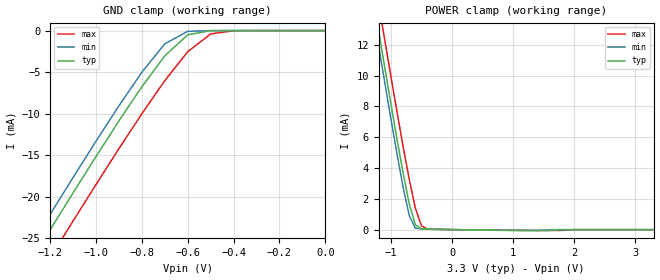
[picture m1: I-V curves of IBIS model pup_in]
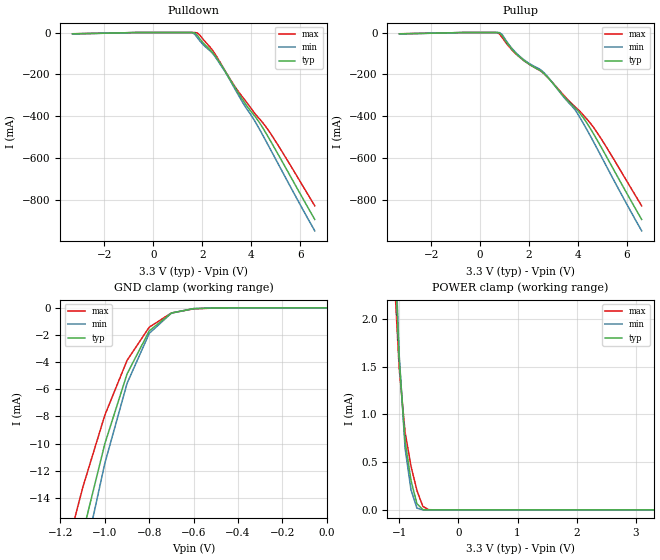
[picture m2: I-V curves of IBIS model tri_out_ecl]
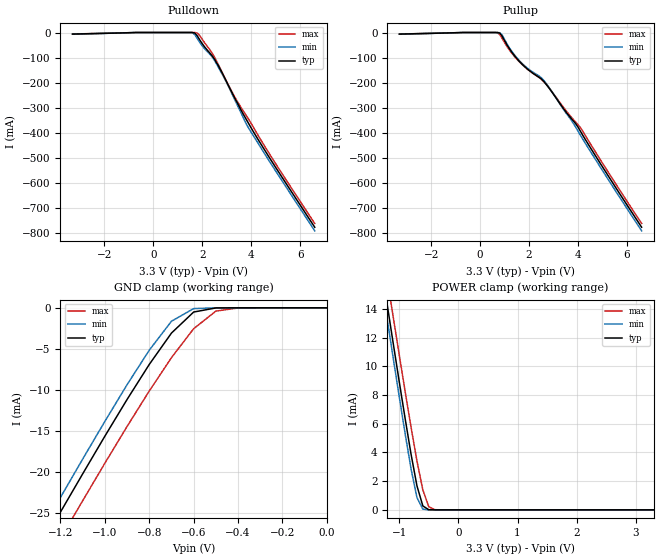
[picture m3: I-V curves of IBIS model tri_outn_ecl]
| IBIS file EG2101CA.ibs
[IBIS ver]   3.2
[File name]   eg2101ca.ibs
[File Rev]   2
[Date]   December 26, 2006
[Source]   Circuits Simulation by HSPICE.
|   Component EG-2101CA
[Component]   EG-2101CA
[Manufacturer]   Epson Toyocom Corp.
[Package]
| variable   typ   min   max
R_pkg   1.04   NA   NA
L_pkg   1.98nH  NA   NA
C_pkg   3.71pF  NA   NA
[Pin]   signal_name   model_name   R_pin   L_pin   C_pin
1   oe   pup_in   NA   NA   NA
4   out   tri_out_ecl   NA   NA   NA
5   outn   tri_outn_ecl   NA   NA   NA
6   vdd   POWER   NA   NA   NA
3   vss   GND   NA   NA   NA
[Diff Pin] inv_pin vdiff   tdelay_typ
4   5   0   0
| Models and submodels in the file (3): pup_in (Input), tri_out_ecl (3-state_ECL), tri_outn_ecl (3-state_ECL)
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|   Model pup_in
[Model]   pup_in
Model_type   Input
C_comp   1.00pF  0.70pF  1.43pF
Vinl = 0.99V | VIL = VCC * 0.3
Vinh = 2.31V | VIH = VCC * 0.7
|   typ   min   max
[Temperature Range]   25.00  0.000  70.00
[Voltage Range]   3.30V  3.00V  3.60V
[POWER Clamp Reference]   3.30V  3.00V  3.60V
[GND Clamp Reference]   0.00V  0.00V  0.00V
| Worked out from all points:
|   GND clamp passes 1 mA (typ) near -0.62 V on its own axis
|   POWER clamp passes 1 mA (typ) near -0.65 V on its own axis
[GND_clamp]
| voltage = voutput
| voltage   I(typ)   I(min)   I(max)
-3.3V     -120.5mA   -118.7mA   -123.7mA
-1.3V     -28.46mA   -26.61mA   -31.84mA
-1.2V     -23.98mA   -22.12mA   -27.37mA
-1.1V     -19.54mA   -17.68mA   -22.92mA
-900mV    -10.87mA   -9.048mA   -14.21mA
-800mV    -6.758mA   -5.013mA   -10.01mA
-700mV    -3.036mA   -1.593mA   -6.026mA
-600mV    -509.4uA   -93.51uA   -2.539mA
-500mV    -21.23uA   -6.595uA   -406.6uA
-400mV    -6.143uA   -5.249uA   -23.62uA
0V        -5.82uA    -5.224uA   -5.655uA
[POWER_clamp]
| voltage = vcc - voutput
| voltage   I(typ)   I(min)   I(max)
-3.3V     64.56mA    63.65mA    66.23mA
-1.3V     15.28mA    14.3mA     17.06mA
-1.2V     12.88mA    11.9mA     14.67mA
-1.1V     10.5mA     9.52mA     12.29mA
-900mV    5.86mA     4.896mA    7.632mA
-800mV    3.66mA     2.731mA    5.38mA
-700mV    1.667mA    901.9uA    3.253mA
-600mV    312.1uA    93.69uA    1.387mA
-500mV    44.06uA    39.07uA    243.8uA
-400mV    28.45uA    30.18uA    33.23uA
1.4V      -59.9uA    -54.53uA   -54.76uA
3.3V      -5.82uA    -5.228uA   -5.652uA
|   Model tri_out_ecl
[Model]   tri_out_ecl
Model_type   3-state_ECL
Polarity   Non-Inverting
Enable   Active-High
C_comp   1.00pF  0.70pF  1.43pF
Vmeas = 1.97V | Vmeas = ( VOH - VOL ) / 2 + VOL
Rref  = 50.0
Vref  = 1.3V  | Vref = vcc - 2V
[Temperature Range]   25.00  0.000  70.00
[Voltage Range]   3.30V  3.00V  3.60V
[POWER Clamp Reference]   3.30V  3.00V  3.60V
[Pullup Reference]   3.30V  3.00V  3.60V
[Pulldown Reference]   3.30V  3.00V  3.60V
[GND Clamp Reference]   0.00V  0.00V  0.00V
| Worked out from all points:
|   GND clamp passes 1 mA (typ) near -0.75 V on its own axis
|   POWER clamp passes 1 mA (typ) near -0.93 V on its own axis
[GND_clamp]
| voltage = voutput
| voltage   I(typ)   I(min)   I(max)
-3.3V     -542.7mA   -569.9mA   -497.4mA
-1.2V     -24.33mA   -27.52mA   -19.57mA
-1.1V     -16.63mA   -18.92mA   -13.25mA
-1V       -10mA      -11.44mA   -7.898mA
-900mV    -4.868mA   -5.562mA   -3.869mA
-800mV    -1.697mA   -1.88mA    -1.427mA
-700mV    -384.8uA   -387.2uA   -376.6uA
-600mV    -62.16uA   -53.48uA   -76.64uA
-500mV    -8.105uA   -5.742uA   -13.19uA
0V        -255.1pA   -231.2pA   -288.8pA
[POWER_clamp]
| voltage = vcc - voutput
| voltage   I(typ)   I(min)   I(max)
-3.3V     100.7mA    114.9mA    80.47mA
-1.1V     3.06mA     3.326mA    2.658mA
-1V       1.575mA    1.627mA    1.486mA
-900mV    717.9uA    644.3uA    812.2uA
-800mV    308.6uA    208.8uA    457.2uA
-700mV    63.92uA    17.64uA    202.1uA
-600mV    2.363uA    311.8nA    35.6uA
-500mV    51.2nA     5.01nA     1.698uA
3.3V      -255.1pA   -28.35nA   -178.4pA
[Pulldown]
| voltage = vcc - voutput
| voltage   I(typ)   I(min)   I(max)
-3.3V     -6.27mA    -6.5mA     -5.99mA
1.5V      -1.431uA   -9.535uA   -138nA
1.7V      -2.193mA   -8.846mA   -105.2uA
1.9V      -29.67mA   -39.67mA   -12.53mA
2.4V      -92.19mA   -96.42mA   -81.15mA
2.7V      -139.8mA   -145.5mA   -136.1mA
3V        -197.2mA   -200mA     -195.4mA
3.5V      -292.9mA   -302.6mA   -285.3mA
3.9V      -362.5mA   -377.4mA   -346mA
4.3V      -423.1mA   -452.9mA   -406.8mA
4.8V      -519mA     -560.2mA   -482.8mA
6.6V      -891.7mA   -946.1mA   -826.8mA
[Pullup]
| voltage = vcc -voutput
| voltage   I(typ)   I(min)   I(max)
-3.3V     -6.33mA    -6.5mA     -6.04mA
600mV     -1.429uA   -178.2nA   -29.67uA
800mV     -2.257mA   -696.2uA   -8.199mA
900mV     -15.26mA   -10.35mA   -23.87mA
1.2V      -65.31mA   -61.67mA   -70.26mA
1.6V      -114.7mA   -111.9mA   -116.7mA
2.6V      -194.8mA   -190.8mA   -195.7mA
3.5V      -315.4mA   -319.4mA   -310.1mA
3.9V      -362.1mA   -372.2mA   -356.4mA
4.3V      -420.7mA   -450.5mA   -404.8mA
4.8V      -516.7mA   -557.9mA   -480.7mA
6.6V      -891.5mA   -945.9mA   -826.5mA
[Ramp]
| variable   typ   min   max
dV/dt_r   481.0m/512.2p  433.4m/517.5p  555.7m/498.7p
dV/dt_f   481.0m/346.7p  433.4m/350.0p  555.7m/355.1p
R_load = 50.00
| End [Model] tri_out_ecl
|   Model tri_outn_ecl
[Model]   tri_outn_ecl
Model_type   3-state_ECL
Polarity   Inverting
Enable   Active-High
C_comp   1.00pF  0.70pF  1.43pF
Vmeas = 1.97V | Vmeas = ( VOH - VOL ) / 2 + VOL
Rref  = 50.0
Vref  = 1.3V  | Vref = vcc - 2V
[Temperature Range]   25.00  0.000  70.00
[Voltage Range]   3.30V  3.00V  3.60V
[POWER Clamp Reference]   3.30V  3.00V  3.60V
[Pullup Reference]   3.30V  3.00V  3.60V
[Pulldown Reference]   3.30V  3.00V  3.60V
[GND Clamp Reference]   0.00V  0.00V  0.00V
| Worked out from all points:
|   GND clamp passes 1 mA (typ) near -0.62 V on its own axis
|   POWER clamp passes 1 mA (typ) near -0.65 V on its own axis
[GND_clamp]
| voltage = voutput
| voltage   I(typ)   I(min)   I(max)
-3.3V     -426.7mA   -431.7mA   -417.9mA
-1.3V     -29.56mA   -27.81mA   -32.77mA
-1.2V     -24.87mA   -23.09mA   -28.11mA
-1.1V     -20.22mA   -18.42mA   -23.49mA
-900mV    -11.16mA   -9.365mA   -14.45mA
-800mV    -6.895mA   -5.161mA   -10.13mA
-700mV    -3.076mA   -1.634mA   -6.065mA
-600mV    -512.6uA   -96.1uA    -2.544mA
-500mV    -16.66uA   -2.257uA   -402.9uA
-400mV    -449nA     -93.48nA   -18.24uA
0V        -152.9pA   -138.2pA   -190.1pA
[POWER_clamp]
| voltage = vcc - voutput
| voltage   I(typ)   I(min)   I(max)
-3.3V     71.52mA    70.86mA    72.74mA
-1.3V     16.91mA    15.92mA    18.68mA
-1.2V     14.24mA    13.23mA    16.05mA
-1.1V     11.59mA    10.56mA    13.43mA
-900mV    6.383mA    5.326mA    8.273mA
-800mV    3.898mA    2.869mA    5.778mA
-700mV    1.679mA    863.7uA    3.412mA
-600mV    270.9uA    47.25uA    1.387mA
-500mV    8.267uA    732nA      215.5uA
-400mV    170.8nA    10.5nA     9.638uA
3.3V      -152.9pA   -5.01nA    -139.4pA
[Pulldown]
| voltage = vcc - voutput
| voltage   I(typ)   I(min)   I(max)
-3.3V     -6.31mA    -6.46mA    -6mA
1.6V      -65.57uA   -573.1uA   -3.823uA
1.7V      -2.193mA   -8.846mA   -105.2uA
1.8V      -14mA      -24.44mA   -2.19mA
2V        -44.44mA   -53.23mA   -27mA
2.4V      -92.19mA   -96.42mA   -81.15mA
2.6V      -122.6mA   -127.7mA   -116.5mA
2.9V      -177.3mA   -181mA     -175.8mA
3.3V      -255.5mA   -261.5mA   -251.6mA
3.9V      -363mA     -381.2mA   -346mA
5V        -537.2mA   -551.3mA   -522.3mA
6.6V      -775.8mA   -790.1mA   -760.8mA
[Pullup]
| voltage = vcc - voutput
| voltage   I(typ)   I(min)   I(max)
-3.3V     -6.36mA    -6.51mA    -6.05mA
600mV     -1.429uA   -178.2nA   -29.67uA
800mV     -2.257mA   -696.2uA   -8.199mA
900mV     -15.26mA   -10.35mA   -23.87mA
1.2V      -65.31mA   -61.67mA   -70.26mA
1.6V      -114.7mA   -111.9mA   -116.7mA
2V        -150.8mA   -147.3mA   -151.5mA
2.6V      -194.8mA   -190.8mA   -195.7mA
3.7V      -339.8mA   -345.9mA   -334.2mA
3.9V      -362.6mA   -376mA     -356.4mA
4.1V      -393.5mA   -409.5mA   -379.2mA
6.6V      -775.5mA   -789.9mA   -760.5mA
[Ramp]
| variable   typ   min   max
dV/dt_r   480.8m/502.1p  433.3m/506.8p  556.0m/486.5p
dV/dt_f   480.8m/347.1p  433.3m/350.3p  556.0m/357.0p
R_load = 50.00
| End [Model] tri_outn_ecl
| End [Component] EG-2101CA
